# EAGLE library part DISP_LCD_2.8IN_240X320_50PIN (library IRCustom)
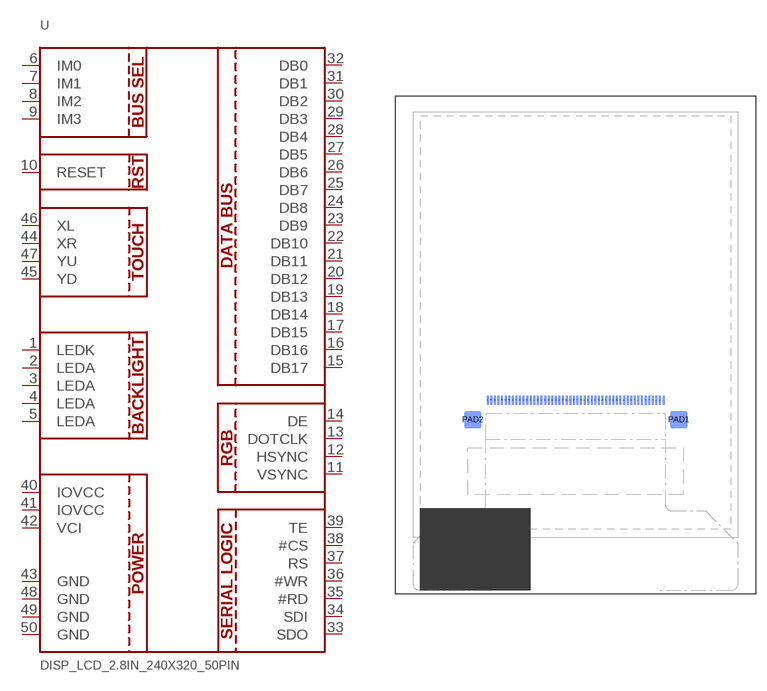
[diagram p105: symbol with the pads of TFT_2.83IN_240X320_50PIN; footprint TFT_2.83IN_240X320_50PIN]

Designator prefix -

## DISP_LCD_2.8IN_240X320_50PIN  [TFT_2.83IN_240X320_50PIN]
1  LEDK
2  LEDA
3  LEDA
4  LEDA
5  LEDA
6  IM0
7  IM1
8  IM2
9  IM3
10  RESET
11  VSYNC
12  HSYNC
13  DOTCLK
14  DE
15  DB17
16  DB16
17  DB15
18  DB14
19  DB13
20  DB12
21  DB11
22  DB10
23  DB9
24  DB8
25  DB7
26  DB6
27  DB5
28  DB4
29  DB3
30  DB2
31  DB1
32  DB0
33  SDO
34  SDI
35  #RD
36  #WR
37  RS
38  #CS
39  TE
40  IOVCC
41  IOVCC
42  VCI
43  GND
44  XR
45  YD
46  XL
47  YU
48  GND
49  GND
50  GND

## Footprint TFT_2.83IN_240X320_50PIN (pad centres in mm)
smd 0.275 x 1.2 bottom: 1 12.25,-10.39; 2 11.75,-10.39; 3 11.25,-10.39; 4 10.75,-10.39; 5 10.25,-10.39; 6 9.75,-10.39; 7 9.25,-10.39; 8 8.75,-10.39; 9 8.25,-10.39; 10 7.75,-10.39; 11 7.25,-10.39; 12 6.75,-10.39; 13 6.25,-10.39; 14 5.75,-10.39; 15 5.25,-10.39; 16 4.75,-10.39; 17 4.25,-10.39; 18 3.75,-10.39; 19 3.25,-10.39; 20 2.75,-10.39; 21 2.25,-10.39; 22 1.75,-10.39; 23 1.25,-10.39; 24 0.75,-10.39; 25 0.25,-10.39; 26 -0.25,-10.39; 27 -0.75,-10.39; 28 -1.25,-10.39; 29 -1.75,-10.39; 30 -2.25,-10.39; 31 -2.75,-10.39; 32 -3.25,-10.39; 33 -3.75,-10.39; 34 -4.25,-10.39; 35 -4.75,-10.39; 36 -5.25,-10.39; 37 -5.75,-10.39; 38 -6.25,-10.39; 39 -6.75,-10.39; 40 -7.25,-10.39; 41 -7.75,-10.39; 42 -8.25,-10.39; 43 -8.75,-10.39; 44 -9.25,-10.39; 45 -9.75,-10.39; 46 -10.25,-10.39; 47 -10.75,-10.39; 48 -11.25,-10.39; 49 -11.75,-10.39; 50 -12.25,-10.39
smd 2.4 x 2.4 bottom: PAD1 14.35,-13.09; PAD2 -14.35,-13.09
